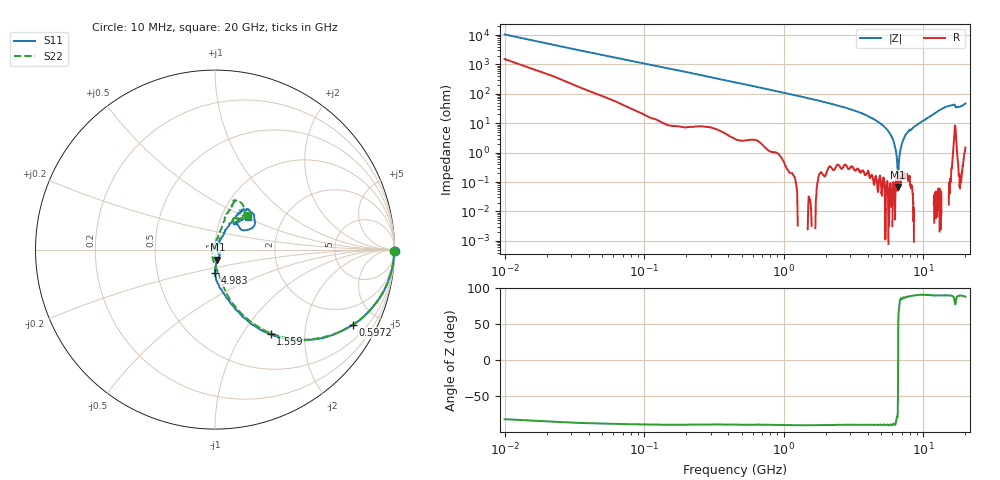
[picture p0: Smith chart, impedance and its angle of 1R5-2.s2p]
!Keysight Technologies,P5008B,MY61100088,A.16.20.02
!Date: Monday, May 27, 2024 14:00:18
!Correction: S11(C  2-Port  )
!S21(C  2-Port  )
!S12(C  2-Port  )
!S22(C  2-Port  )
!S2P File: Measurements: S11, S21, S12, S22:
# Hz S  dB  R 50
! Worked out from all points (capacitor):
!   1601 points, 10 MHz to 20 GHz, reference 50 ohm
!   read as one part in series: C = 1.45 pF near 110 MHz
!   lowest |Z| = 68.2 mohm at 6.594 GHz (marker M1)
!   series resonance near 6.592 GHz, so ESL is about 400 pH
!   S11 on the Smith chart (normalised r, x): 10 MHz: open; 597.2 MHz: 1.02, -3.67; 1.559 GHz: 0.97, -1.35; 4.983 GHz: 0.96, -0.26; 20 GHz: 1.34, +0.52
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1e7  0.01 -0.6  -40.39 81.1  -40.39 81.1  -0.02 -0.5
1.224438e8  -0.08 -6.5  -19.02 82.7  -19.03 82.7  -0.07 -6.5
1.974062e8  -0.17 -10.4  -15.13 79.0  -15.14 79.0  -0.16 -10.2
3.59825e8  -0.49 -18.2  -10.16 70.8  -10.17 70.8  -0.49 -18.2
5.972062e8  -1.15 -28.5  -6.52 60.6  -6.54 60.6  -1.17 -28.5
1.559225e9  -4.97 -56.7  -1.65 33.6  -1.66 33.6  -4.94 -55.9
3.345831e9  -11.53 -77.3  -0.31 12.9  -0.32 12.9  -11.64 -74.7
4.982512e9  -17.72 -90.4  -0.07 3.2  -0.08 3.2  -17.77 -82.0
6.594206e9  -24.80 -76.8  0.01 -3.2  0.00 -3.2  -24.95 -102.2
6.681662e9  -25.19 -74.0  0.02 -3.5  0.00 -3.5  -25.51 -101.6
7.718644e9  -29.67 -40.4  0.03 -6.8  0.02 -6.8  -32.50 -136.7
8.268369e9  -30.33 -46.3  0.03 -8.5  0.02 -8.5  -33.27 -138.8
9.242881e9  -37.37 -24.6  0.05 -11.3  0.03 -11.3  -40.16 175.6
9.555225e9  -39.87 -4.7  0.05 -12.2  0.04 -12.1  -40.69 149.8
1.0005e10  -35.28 42.5  0.05 -13.4  0.04 -13.4  -35.77 101.5
1.131684e10  -23.04 64.3  0.03 -17.2  0.02 -17.1  -23.67 76.3
1.334083e10  -14.33 58.8  -0.10 -22.9  -0.11 -22.8  -14.41 72.2
1.474013e10  -11.36 55.9  -0.26 -26.8  -0.26 -26.7  -11.37 68.4
1.667666e10  -11.16 37.3  -0.70 -31.5  -0.71 -31.5  -10.51 60.5
1.706397e10  -14.80 39.5  -0.55 -27.6  -0.57 -27.5  -13.25 53.5
1.835082e10  -15.09 53.0  -0.09 -33.2  -0.10 -33.2  -14.91 56.8
2e10  -11.71 44.4  -0.36 -39.8  -0.37 -39.8  -11.66 47.2
